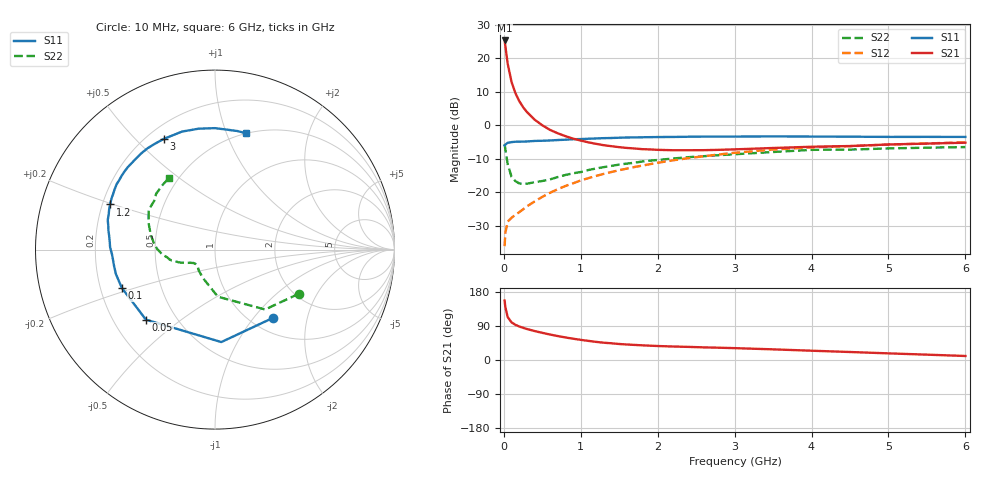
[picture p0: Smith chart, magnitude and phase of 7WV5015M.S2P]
! Infineon Technologies  Discrete & RF Semiconductors
! BFS17W
! Si NPN RF Bipolar Junction Transistor in SOT323
! VCE = 0.5 V  IC = 15 mA
! Common Emitter S-Parameters:  August  1999
# GHz  S  MA  R  50
!  f  S11  S21  S12  S22
! GHz  MAG  ANG  MAG  ANG  MAG  ANG  MAG  ANG
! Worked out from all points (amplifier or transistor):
!   36 points, 10 MHz to 6 GHz, reference 50 ohm
!   highest |S21| = 25.3 dB at 10 MHz (marker M1)
!   |S21| within 3 dB of that: start of sweep to 27.4 MHz
!   unconditionally stable (mu >= 1): 40.91 MHz to end of sweep
!   at 250 MHz: K = 3.21, MAG = 7.3 dB, |S12| = -25.1 dB
!   at 1.4 GHz: K = 2.90, MAG = -3.7 dB, |S12| = -13.9 dB
!   at 6 GHz: K = 1.16, MAG = -2.5 dB, |S12| = -5.0 dB
!   S11 on the Smith chart (normalised r, x): 10 MHz: 1.24, -1.26; 50 MHz: 0.34, -0.38; 100 MHz: 0.29, -0.18; 1.2 GHz: 0.23, +0.20; 3 GHz: 0.26, +0.61; 6 GHz: 0.50, +1.17
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0.01  0.4987 -49.8  18.38 156.9  0.0158 67.3  0.5268 -27.9
0.02  0.5163 -86.1  15.1 139.1  0.0252 52.7  0.4351 -50.1
0.05  0.5482 -134.6  8.273 113.3  0.0367 34.5  0.263 -86.5
0.1  0.5614 -157.7  4.436 99.3  0.0418 32.1  0.171 -113.7
0.15  0.5688 -166.3  3.022 92.8  0.0462 36.8  0.1474 -127.8
0.2  0.5699 -171.2  2.299 88.5  0.0507 40.7  0.1364 -134.8
0.25  0.5717 -174.9  1.867 85.0  0.0559 44.5  0.1337 -140.7
0.3  0.574 -177.1  1.577 81.9  0.0619 47.8  0.1346 -143.7
0.4  0.5847 178.6  1.213 76.4  0.0733 52.7  0.142 -148.5
0.5  0.5883 175.6  1.002 71.7  0.0859 55.7  0.1479 -149.8
0.6  0.5941 172.8  0.855 67.2  0.0986 57.5  0.1561 -152.0
0.8  0.6099 167.2  0.689 59.5  0.1245 59.3  0.1818 -156.0
1.1  0.6308 159.2  0.557 50.4  0.1633 59.6  0.2157 -160.9
1.2  0.6365 156.7  0.529 47.8  0.1761 59.4  0.2274 -163.1
1.6  0.6584 146.2  0.46 40.9  0.2263 56.9  0.2686 -170.5
2.2  0.6703 132.2  0.425 35.6  0.3006 51.7  0.32 179.8
3  0.6795 114.9  0.438 31.3  0.3897 42.7  0.3703 166.0
3.5  0.6828 105.6  0.459 28.1  0.4355 36.6  0.3999 157.9
4  0.6798 97.7  0.479 24.5  0.4687 30.4  0.4306 149.2
4.5  0.6767 90.1  0.491 21.1  0.4885 25.3  0.4344 141.2
5.5  0.6722 79.3  0.534 14.1  0.5362 16.8  0.4638 129.1
6  0.6709 75.1  0.55 10.6  0.5593 12.6  0.4739 122.7
